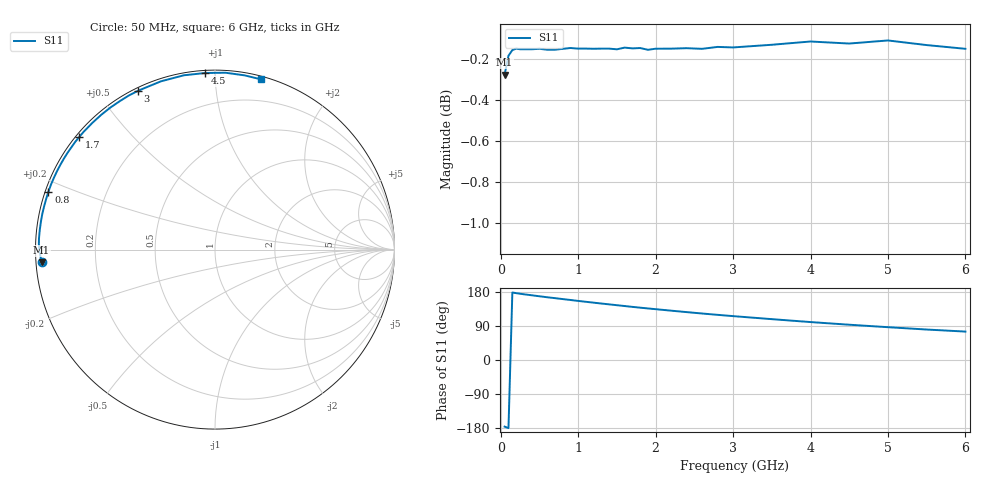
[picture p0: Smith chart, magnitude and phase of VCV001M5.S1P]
! Infineon Technologies  Discrete & RF Semiconductors
! BBY 56-03
! Si Tuning Diode in SOD323
! VR =
! S-Parameters:  June  1999
# GHz  S  MA  R  50
!  f  S11
! GHz  MAG  ANG
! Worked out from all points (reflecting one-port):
!   34 points, 50 MHz to 6 GHz, reference 50 ohm
!   lowest |S11| = -0.3 dB at 50 MHz (marker M1), VSWR 62.51, Z = 0.801 - j1.83 ohm
!   phase of S11 starts at -176 deg and turns -109 deg over the sweep
!   S11 on the Smith chart (normalised r, x): 50 MHz: 0.02, -0.04; 800 MHz: 0.01, +0.17; 1.7 GHz: 0.01, +0.36; 3 GHz: 0.01, +0.63; 4.5 GHz: 0.01, +0.95; 6 GHz: 0.02, +1.30
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0.05  0.9685 -175.8
0.1  0.9788 -179.7
0.15  0.9819 178.1
0.2  0.9827 176.4
0.3  0.9823 173.4
0.5  0.9826 168.2
0.6  0.9821 165.6
0.8  0.9826 160.8
0.9  0.983 158.4
1  0.9827 155.9
1.2  0.9826 151.3
1.3  0.9827 149.0
1.4  0.9827 146.8
1.6  0.9832 142.4
1.7  0.9828 140.2
1.8  0.983 138.1
2  0.9826 134.1
2.2  0.9827 130.2
2.4  0.9829 126.4
2.6  0.9826 122.7
2.8  0.9836 119.2
3  0.9833 115.8
3.5  0.9848 107.8
4  0.9866 100.1
4.5  0.9855 93.1
5  0.9872 86.6
5.5  0.9846 80.4
6  0.9826 75.0
